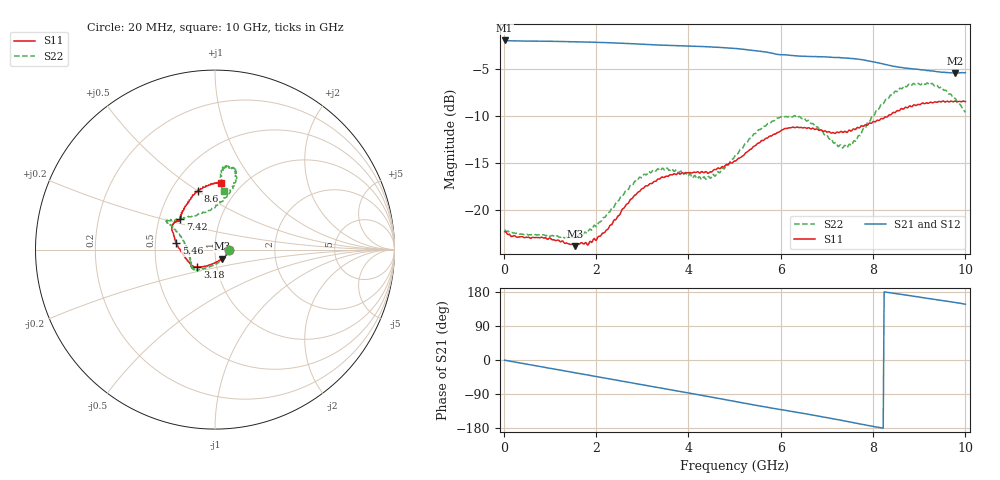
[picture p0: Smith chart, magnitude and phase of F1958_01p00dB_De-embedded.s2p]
! Integrated Device Technology
! Corporate Headquarters
! 6024 Silver Creek Valley Road
! San Jose, CA 95138  USA
! Phone:  1-408-284-8200
! Toll Free:  1-800-223-1366
! Webpage:  http://www.idt.com/
! Timing and RF Division
! 515 Groton Road, Suite 102
! Westford, MA 01886-6024
! Device:  F1958
! Description: 7-bit 0.25 dB Digital Step Attenuator
! Frequency:  0.001 -  6.000 GHz
! Package:  4x4 mm Thin QFN Plastic Package: 24 pin
! Ports:  2 RF, 12 DC
!  Pin  1  = D0
!  Pin  2  = VDD
!  Pin  3  = VMODE
!  Pin  4  = GND
!  Pin  5  = RF1  =  Port 1
!  Pin  6  = GND
!  Pin  7  = GND
!  Pin  8  = GND
!  Pin  9  = GND
!  Pin 10  = GND
!  Pin 11  = GND
!  Pin 12  = GND
!  Pin 13  = GND
!  Pin 14  = RF2  =  Port 2
!  Pin 15  = GND
!  Pin 16  = LE
!  Pin 17  = CLK
!  Pin 18  = DATA
!  Pin 19  = D6
!  Pin 20  = D5
!  Pin 21  = D4
!  Pin 22  = D3
!  Pin 23  = D2
!  Pin 24  = D1
! State:  4
! Atten State:  1.00 dB
! Voltage:  +3.30 Volts
! Current:  0.257 mA
! Data:  The device was measured on a F1958 evaluation board which has
!  individual transmission lines to the RF pins.  Data was collected
!  using a calibrated network analyzer.  The evaluation board was
!  de-embedded using Automatic Fixture Removal (AFR).
!  The reference plane is the edge of the package pin.
! Misc:
!  Action Tracker AT0419
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# GHz S dB R 50
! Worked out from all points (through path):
!   500 points, 20 MHz to 10 GHz, reference 50 ohm
!   highest |S21| = -2.02 dB at 20 MHz (marker M1); lowest = -5.5 dB at 9.78 GHz (marker M2)
!   group delay of S21, straight-line fit = 59.9 ps
!   lowest |S11| = -23.9 dB at 1.54 GHz (marker M3), VSWR 1.14, Z = 53.9 - j5.41 ohm
!   |S11| at or under -10 dB: start of sweep to 8.335 GHz
!   |S22| runs from -23.0 to -6.5 dB; largest |S21 - S12| = 0.002
!   S11 on the Smith chart (normalised r, x): 20 MHz: 1.16, -0.01; 3.18 GHz: 0.81, -0.16; 5.46 GHz: 0.64, +0.05; 7.42 GHz: 0.64, +0.23; 8.6 GHz: 0.67, +0.50; 10 GHz: 0.80, +0.70
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0.02  -22.37 -1.9  -2.02 -0.6  -2.02 -0.6  -22.16 -2.2
0.82  -22.94 -18.2  -2.10 -17.8  -2.10 -17.8  -22.70 -23.8
1.54  -23.90 -51.5  -2.16 -33.5  -2.16 -33.4  -22.85 -61.5
1.7  -23.54 -61.3  -2.18 -36.8  -2.17 -36.8  -22.76 -71.2
2.22  -22.21 -96.0  -2.25 -48.2  -2.24 -48.1  -20.63 -101.8
2.78  -18.84 -124.4  -2.36 -60.5  -2.35 -60.6  -17.44 -125.0
3.18  -17.24 -135.4  -2.47 -69.3  -2.46 -69.3  -16.09 -134.5
3.36  -16.75 -138.1  -2.51 -73.1  -2.51 -73.2  -15.74 -137.6
4.42  -16.15 -151.7  -2.68 -96.1  -2.69 -96.2  -16.51 -172.0
5.02  -14.83 -172.5  -2.87 -109.6  -2.88 -109.6  -14.17 161.4
5.46  -13.18 169.9  -3.11 -119.4  -3.12 -119.4  -11.91 153.1
5.98  -11.72 156.5  -3.53 -130.4  -3.54 -130.4  -10.20 149.9
6.38  -11.26 148.5  -3.67 -138.7  -3.69 -138.6  -10.16 148.3
6.68  -11.36 144.3  -3.73 -144.9  -3.75 -144.8  -10.85 144.2
7.22  -11.76 140.6  -3.84 -157.0  -3.85 -156.9  -13.12 121.5
7.42  -11.77 138.6  -3.90 -161.7  -3.90 -161.6  -13.33 106.7
7.64  -11.37 134.1  -3.98 -166.9  -3.98 -166.9  -12.67 90.5
8.34  -9.97 115.0  -4.65 177.8  -4.65 177.8  -8.15 73.0
8.6  -9.30 106.2  -4.88 173.2  -4.89 173.2  -7.12 75.4
9.26  -8.60 89.9  -5.26 161.2  -5.26 161.2  -6.61 82.5
9.78  -8.46 84.8  -5.48 151.8  -5.50 151.8  -8.19 84.8
10  -8.51 85.0  -5.44 147.1  -5.47 147.2  -9.65 81.7
